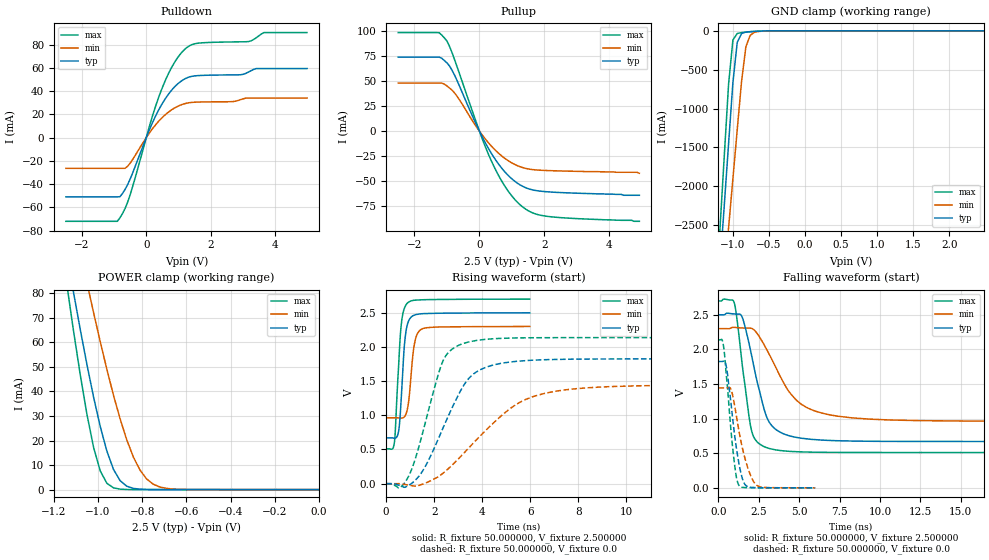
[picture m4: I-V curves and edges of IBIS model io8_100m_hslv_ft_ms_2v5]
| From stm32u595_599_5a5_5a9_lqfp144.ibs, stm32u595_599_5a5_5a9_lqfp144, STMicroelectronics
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|   Model io8_100m_hslv_ft_ms_2v5
[Model]  io8_100m_hslv_ft_ms_2v5
Model_type I/O
Polarity   Non-Inverting
Enable   Active-Low
Vinl =   0.750000V
Vinh =   1.750000V
Vmeas =  1.250000V
Cref =   50.000000pF
Rref =   100.000000M
Vref =   0.0V
C_comp   3.340900pF   3.338500pF   3.380300pF
[Temperature Range]   25.000000   0.140000k   -40.000000
[Pullup Reference]   2.500000V   2.300000V   2.700000V
[Pulldown Reference]   0.0V   0.0V   0.0V
[POWER Clamp Reference]   2.500000V   2.300000V   2.700000V
[GND Clamp Reference]   0.0V   0.0V   0.0V
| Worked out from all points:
|   slope of the pulldown table from 0 to 0.375 V, typ, clamps not added: 16.1 ohm
|   slope of the pullup table from 0 to 0.375 V, typ, clamps not added: 16.6 ohm
|   GND clamp passes 1 mA (typ) near -0.50 V on its own axis
|   POWER clamp passes 1 mA (typ) near -0.86 V on its own axis
|   rising waveform, R_fixture 50.000000, V_fixture 2.500000: 20-80 % time 200ps typ, 226ps min, 206ps max; typ from 0.67 V to 2.5 V
|   rising waveform, R_fixture 50.000000, V_fixture 0.0: 20-80 % time 1.48ns typ, 2.6ns min, 1ns max; typ from 0 V to 1.82 V
|   falling waveform, R_fixture 50.000000, V_fixture 2.500000: 20-80 % time 1.12ns typ, 2.1ns min, 708ps max; typ from 2.5 V to 0.67 V
|   falling waveform, R_fixture 50.000000, V_fixture 0.0: 20-80 % time 606ps typ, 791ps min, 495ps max; typ from 1.82 V to 0 V
[Pulldown]
|Voltage   I(typ)   I(min)   I(max)
-2.5V     -51mA      -26.45mA   -72.04mA
-900mV    -51mA      -26.45mA   -72.04mA
-820mV    -50.89mA   -26.45mA   -69.09mA
-500mV    -35.59mA   -21.93mA   -49.09mA
140mV     9.489mA    5.639mA    13.76mA
460mV     27.5mA     16.24mA    40.22mA
860mV     43.07mA    25.18mA    63.88mA
1.26V     51.38mA    29.65mA    77.49mA
1.66V     53.45mA    30.63mA    81.42mA
3.18V     56.44mA    34.01mA    82.68mA
3.66V     59.44mA    34.01mA    90.42mA
5V        59.44mA    34.01mA    90.42mA
[Pullup]
|Voltage   I(typ)   I(min)   I(max)
-2.5V     74.06mA    48.12mA    98.58mA
-1.24V    74.06mA    48.12mA    98.43mA
-1V       68.25mA    45.17mA    90.14mA
-840mV    60.72mA    41mA       78.19mA
-680mV    49.98mA    34.51mA    63.59mA
-40mV     2.737mA    1.848mA    3.643mA
360mV     -21.77mA   -14.61mA   -29.22mA
840mV     -42.69mA   -28.49mA   -57.8mA
1.32V     -54.89mA   -36.24mA   -75.42mA
1.64V     -58.66mA   -38.36mA   -81.62mA
2.12V     -60.6mA    -39.33mA   -85.19mA
4.92V     -64mA      -42mA      -90mA
[GND_clamp]
|Voltage   I(typ)   I(min)   I(max)
-2.5V     -9.446A    -9.524A    -9.146A
-1.18V    -3.045A    -3.8A      -2.552A
-1.12V    -2.248A    -3.166A    -1.614A
-1.06V    -1.452A    -2.533A    -685.3mA
-1V       -665mA     -1.901A    -117.9mA
-940mV    -148mA     -1.272A    -34.32mA
-880mV    -35.13mA   -651.5mA   -22.79mA
-820mV    -16mA      -203.9mA   -17.07mA
-760mV    -10.46mA   -56.88mA   -12.26mA
-700mV    -7.068mA   -18.52mA   -8.146mA
-400mV    -103.3uA   -375.9uA   -42.12uA
2.48V     0A         14.84nA    0A
[POWER_clamp]
|Voltage   I(typ)   I(min)   I(max)
-2.49V    881mA      773.1mA    1.07A
-1.14V    95.25mA    122.7mA    82.82mA
-1.11V    79.9mA     109.7mA    64.14mA
-1.05V    50.87mA    84.26mA    30.57mA
-1.02V    37.63mA    72.04mA    17.17mA
-990mV    25.71mA    60.25mA    7.621mA
-930mV    8.217mA    38.43mA    713.9uA
-900mV    3.624mA    28.77mA    182.8uA
-840mV    490.7uA    13.24mA    11.35uA
-780mV    56.55uA    4.324mA    699nA
-660mV    716.5nA    226uA      9.775nA
0V        0A         19.49nA    0A
[Ramp]
| variable   typ   min   max
dV/dt_r  1.09512/1.47286n   0.86586/2.59819n   1.28196/1.00206n
dV/dt_f  1.09811/1.11749n   0.80212/2.09985n   1.31360/0.70718n
R_load = 50.000000
[Rising Waveform]
R_fixture= 50.000000
V_fixture= 2.500000
V_fixture_min= 2.300000
V_fixture_max= 2.700000
|time   V(typ)   V(min)   V(max)
0s        669.7mV    963.1mV    510.6mV
336.3ps   665.5mV    963.3mV    586.3mV
384.4ps   666.8mV    963.3mV    793.7mV
516.5ps   764.5mV    962.6mV    1.71V
648.6ps   1.37V      960mV      2.384V
756.8ps   2.008V     978mV      2.563V
876.9ps   2.318V     1.079V     2.639V
1.177ns   2.467V     2.043V     2.684V
1.453ns   2.485V     2.257V     2.69V
5.982ns   2.5V       2.3V       2.7V
[Rising Waveform]
R_fixture= 50.000000
V_fixture= 0.0
V_fixture_min= 0.0
V_fixture_max= 0.0
|time   V(typ)   V(min)   V(max)
0s        -92.07uV   -36.94uV   -134.1uV
700.7ps   -45.98mV   -5.894mV   -17.85mV
1.051ns   990.9uV    -28.46mV   199.5mV
1.351ns   102.5mV    -27.51mV   525.2mV
2.402ns   841.2mV    162.3mV    1.822V
3.403ns   1.523V     508.3mV    2.07V
4.204ns   1.709V     798.9mV    2.114V
5.506ns   1.792V     1.177V     2.133V
7.558ns   1.82V      1.376V     2.136V
24.92ns   1.825V     1.443V     2.137V
[Falling Waveform]
R_fixture= 50.000000
V_fixture= 2.500000
V_fixture_min= 2.300000
V_fixture_max= 2.700000
|time   V(typ)   V(min)   V(max)
0s        2.5V       2.3V       2.7V
951ps     2.512V     2.318V     2.689V
1.101ns   2.511V     2.316V     2.514V
1.451ns   2.475V     2.31V      1.812V
2.052ns   1.909V     2.304V     821.2mV
2.953ns   1.042V     2.012V     583.3mV
3.604ns   834.3mV    1.713V     546.4mV
4.755ns   731.8mV    1.283V     523.2mV
6.657ns   687.1mV    1.066V     513mV
24.92ns   669.7mV    963.1mV    510.6mV
[Falling Waveform]
R_fixture= 50.000000
V_fixture= 0.0
V_fixture_min= 0.0
V_fixture_max= 0.0
|time   V(typ)   V(min)   V(max)
0s        1.825V     1.443V     2.137V
264.3ps   1.826V     1.443V     2.107V
468.5ps   1.773V     1.443V     1.668V
732.7ps   1.307V     1.442V     936.4mV
936.9ps   878.8mV    1.267V     451mV
1.105ns   580.4mV    1.043V     160.2mV
1.261ns   358.4mV    829.3mV    37.44mV
1.646ns   46.78mV    419.7mV    4.139mV
2.39ns    3.152mV    33.5mV     1.649mV
5.982ns   -92.07uV   -36.94uV   -134.1uV
